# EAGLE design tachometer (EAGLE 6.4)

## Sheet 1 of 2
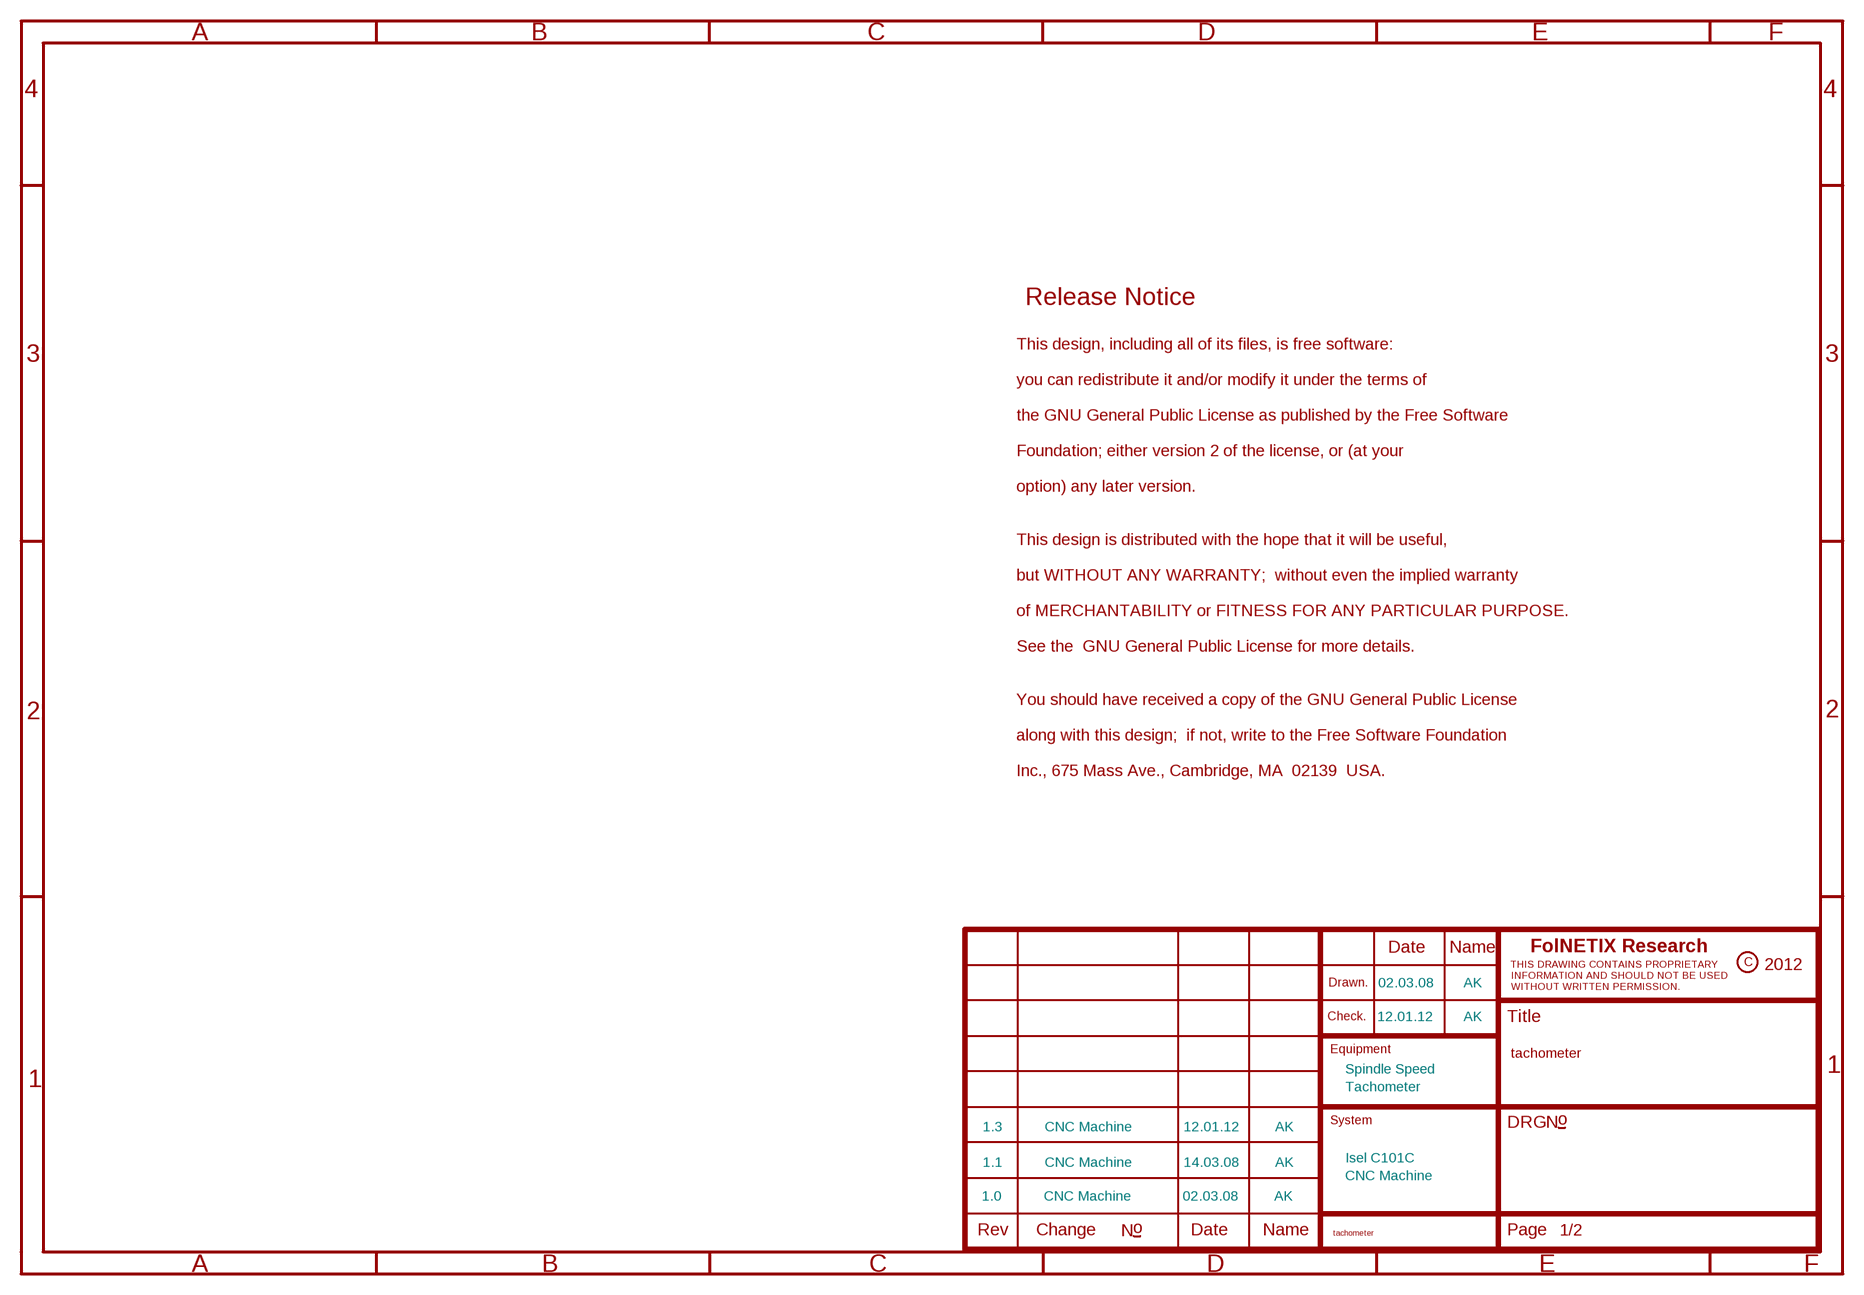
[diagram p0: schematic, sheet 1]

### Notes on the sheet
- 02.03.08 | AK
- 12.01.12 | AK
- Spindle Speed
- Tachometer
- 1.3 | CNC Machine | 12.01.12 | AK
- Isel C101C
- 1.1 | CNC Machine | 14.03.08 | AK
- CNC Machine
- 1.0 | CNC Machine | 02.03.08 | AK

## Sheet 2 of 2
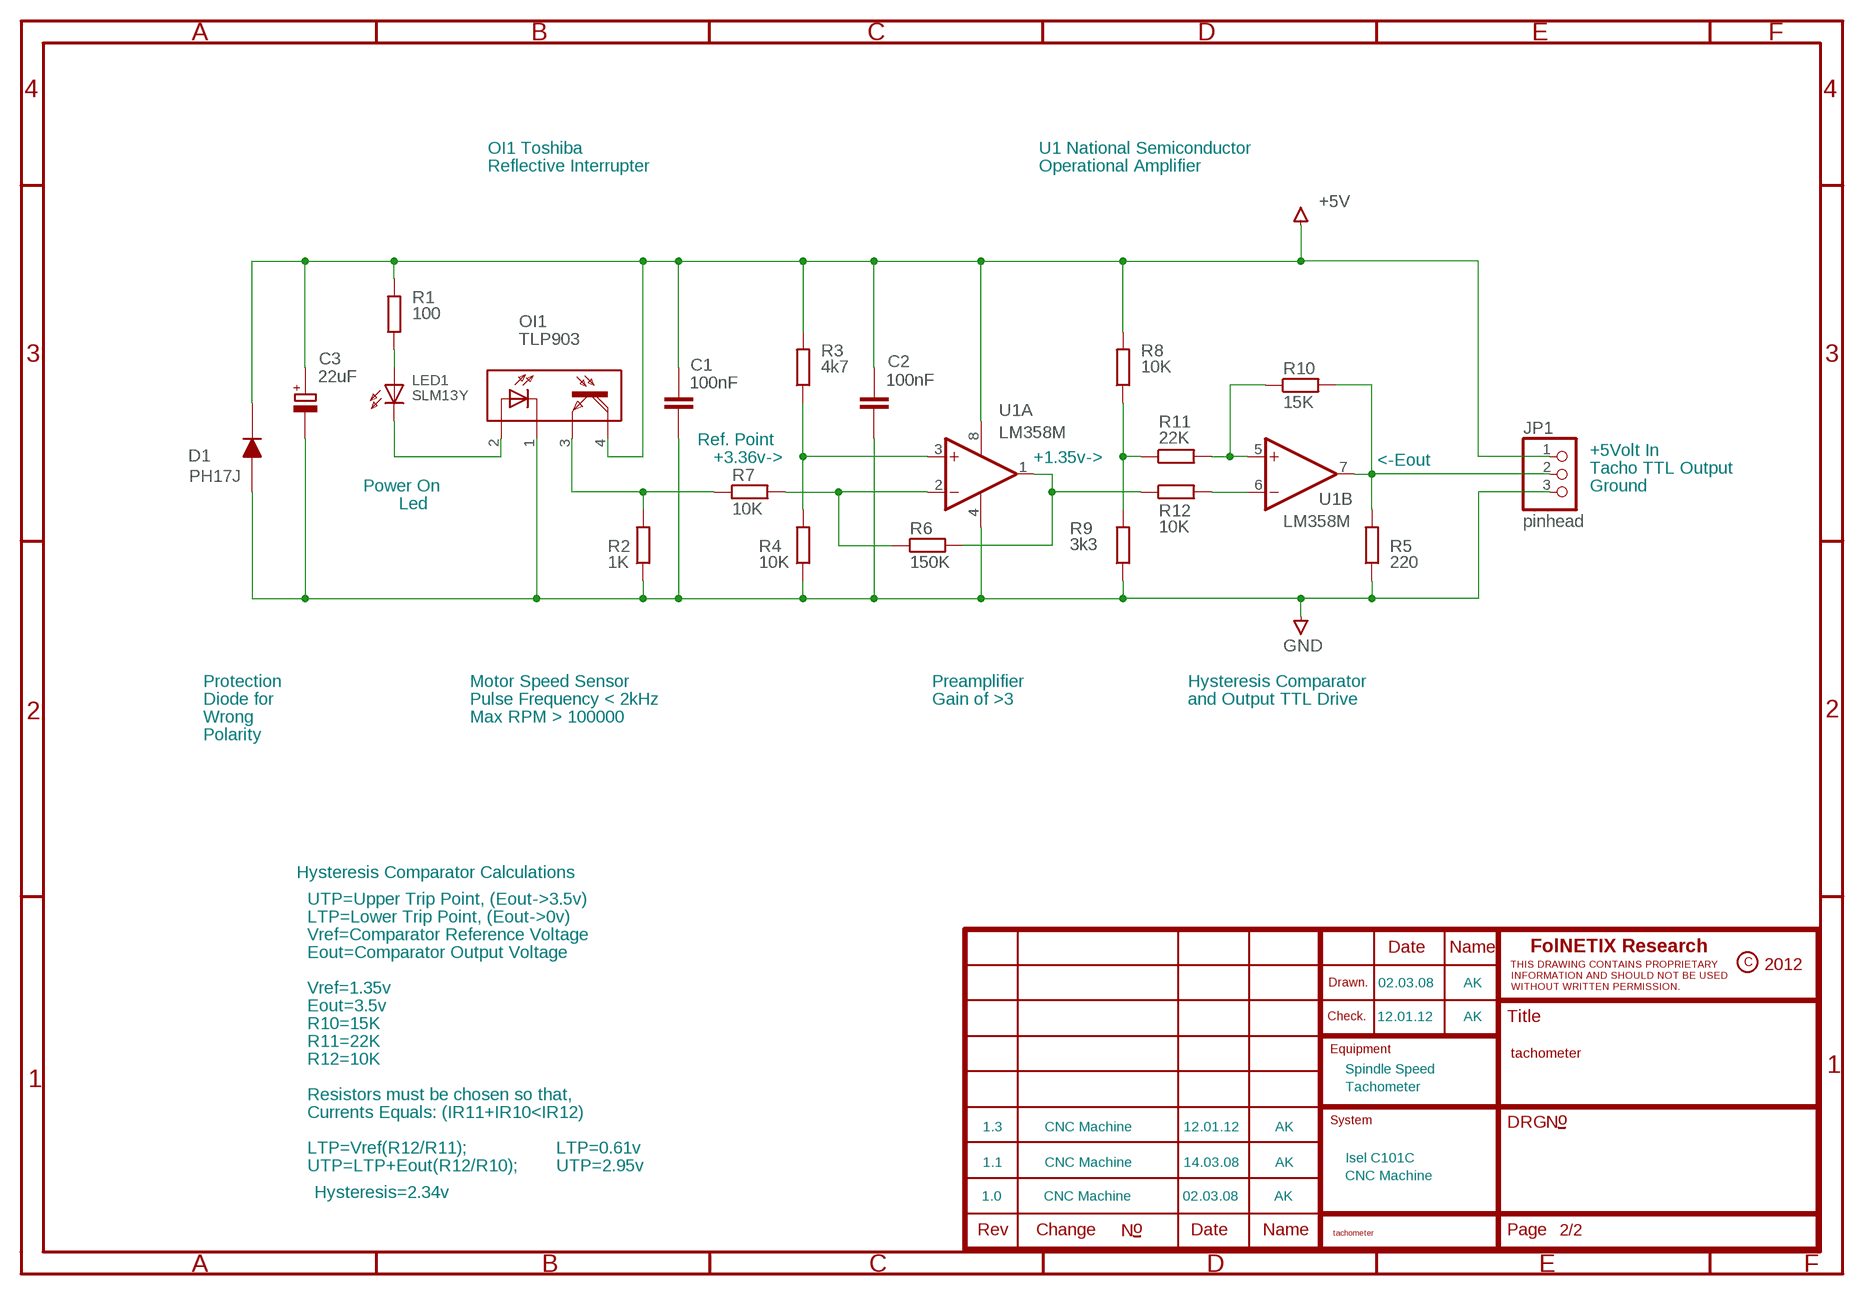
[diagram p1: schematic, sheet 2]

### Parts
C1  100nF  CAPACITOR_0603  [CAPC1608X92N]
C2  100nF  CAPACITOR_0603  [CAPC1608X92N]
C3  22uF  POLARISED_B_CASE  [CAPMP3528X210N]
D1  PH17J  [MELF]
JP1  pinhead  PINHD-1X3M  [1X03M]
LED1  SLM13Y  [SOT23_LED]
OI1  TLP903  [GAP-1E]
R1  100  RESISTOR_0603  [RESC1608X55N]
R2  1K  RESISTOR_0603  [RESC1608X55N]
R3  4k7  RESISTOR_0603  [RESC1608X55N]
R4  10K  RESISTOR_0603  [RESC1608X55N]
R5  220  RESISTOR_0603  [RESC1608X55N]
R6  150K  RESISTOR_0603  [RESC1608X55N]
R7  10K  RESISTOR_0603  [RESC1608X55N]
R8  10K  RESISTOR_0603  [RESC1608X55N]
R9  3k3  RESISTOR_0603  [RESC1608X55N]
R10  15K  RESISTOR_0603  [RESC1608X55N]
R11  22K  RESISTOR_0603  [RESC1608X55N]
R12  10K  RESISTOR_0603  [RESC1608X55N]
U1  LM358M  [SO8]

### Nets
+5V: C1.2 C2.2 C3.+ D1.2(C) JP1.1 OI1.4(TC) R1.2 R3.2 R8.2 U1.8(A:V+)
GND: C1.1 C2.1 C3.- D1.1(A1) JP1.3 OI1.1(LC) R2.1 R4.1 R5.1 R9.1 U1.4(A:V-)
N$1: LED1.3(K) OI1.2(LA)
N$2: OI1.3(TE) R2.2 R7.1
N$3: R3.1 R4.2 U1.3(A:+IN)
N$4: LED1.1(A) R1.1
N$6: JP1.2 R5.2 R10.2 U1.7(B:OUT)
N$7: R6.2 R12.1 U1.1(A:OUT)
N$8: R6.1 R7.2 U1.2(A:-IN)
N$9: R8.1 R9.2 R11.1
N$10: R10.1 R11.2 U1.5(B:+IN)
N$11: R12.2 U1.6(B:-IN)

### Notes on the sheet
- OI1 Toshiba | U1 National Semiconductor
- Reflective Interrupter | Operational Amplifier
- Ref. Point
- +5Volt In
- +3.36v-> | +1.35v-> | <-Eout
- Tacho TTL Output
- Power On | Ground
- Led
- Protection | Motor Speed Sensor | Preamplifier | Hysteresis Comparator
- Diode for | Pulse Frequency < 2kHz | Gain of >3 | and Output TTL Drive
- Wrong | Max RPM > 100000
- Polarity
- Hysteresis Comparator Calculations
- UTP=Upper Trip Point, (Eout->3.5v)
- LTP=Lower Trip Point, (Eout->0v)
- Vref=Comparator Reference Voltage
- Eout=Comparator Output Voltage
- 02.03.08 | AK
- Vref=1.35v
- Eout=3.5v
- 12.01.12 | AK
- R10=15K
- R11=22K
- R12=10K
- Spindle Speed
- Tachometer
- Resistors must be chosen so that,
- Currents Equals: (IR11+IR10<IR12)
- 1.3 | CNC Machine | 12.01.12 | AK
- LTP=Vref(R12/R11); | LTP=0.61v
- Isel C101C
- 1.1 | CNC Machine | 14.03.08 | AK
- UTP=LTP+Eout(R12/R10); | UTP=2.95v
- CNC Machine
- Hysteresis=2.34v | 1.0 | CNC Machine | 02.03.08 | AK

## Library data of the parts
C1 C2 = ipc-7351-capacitor:CAPACITOR_
C3 = ipc-7351-capacitor:POLARISED_
D1 = diode_mpad:PH17J
JP1 = pinhead_extra:PINHD-1X3: PIN HEADER
LED1 = user1:SLM13Y
OI1 = misc_opto:TLP903
R1-R12 = ipc-7351-resistor:RESISTOR_
U1 = user1:LM358M

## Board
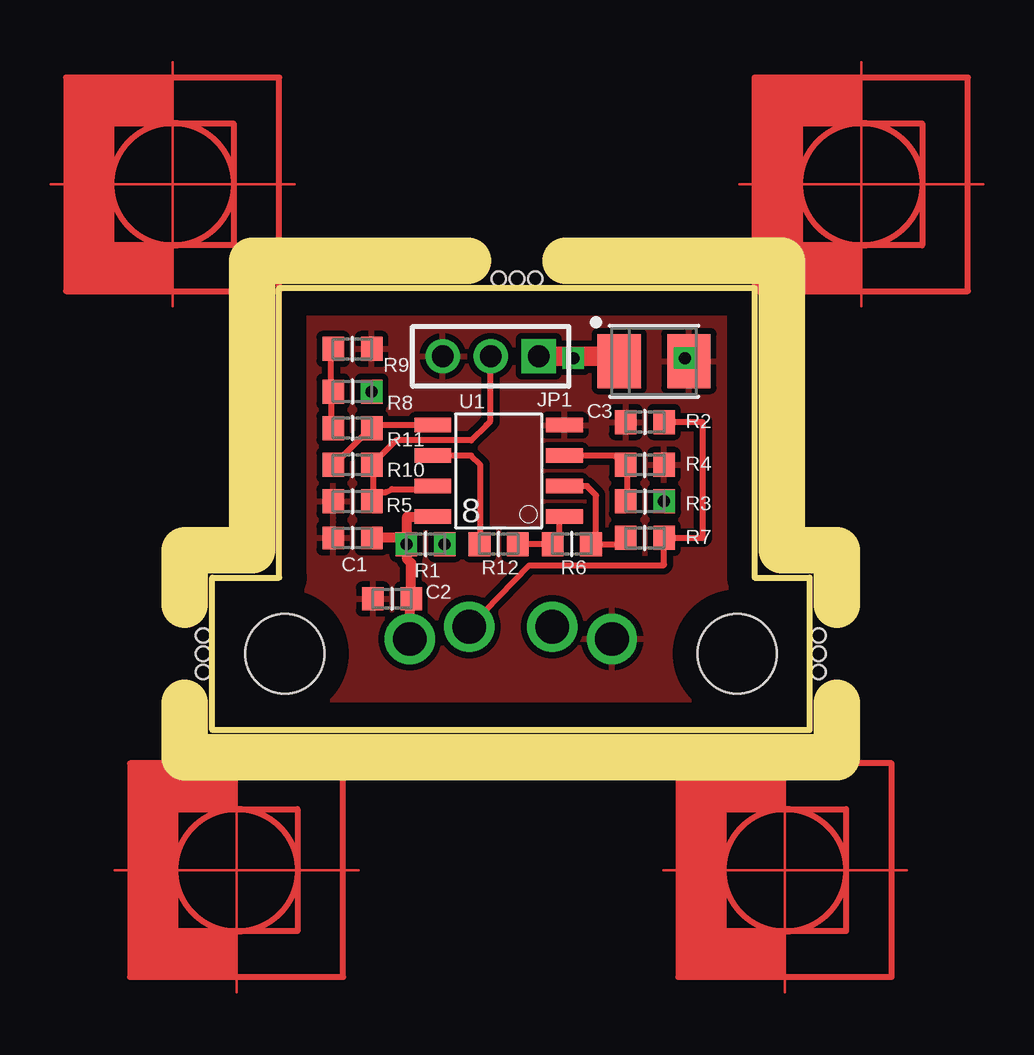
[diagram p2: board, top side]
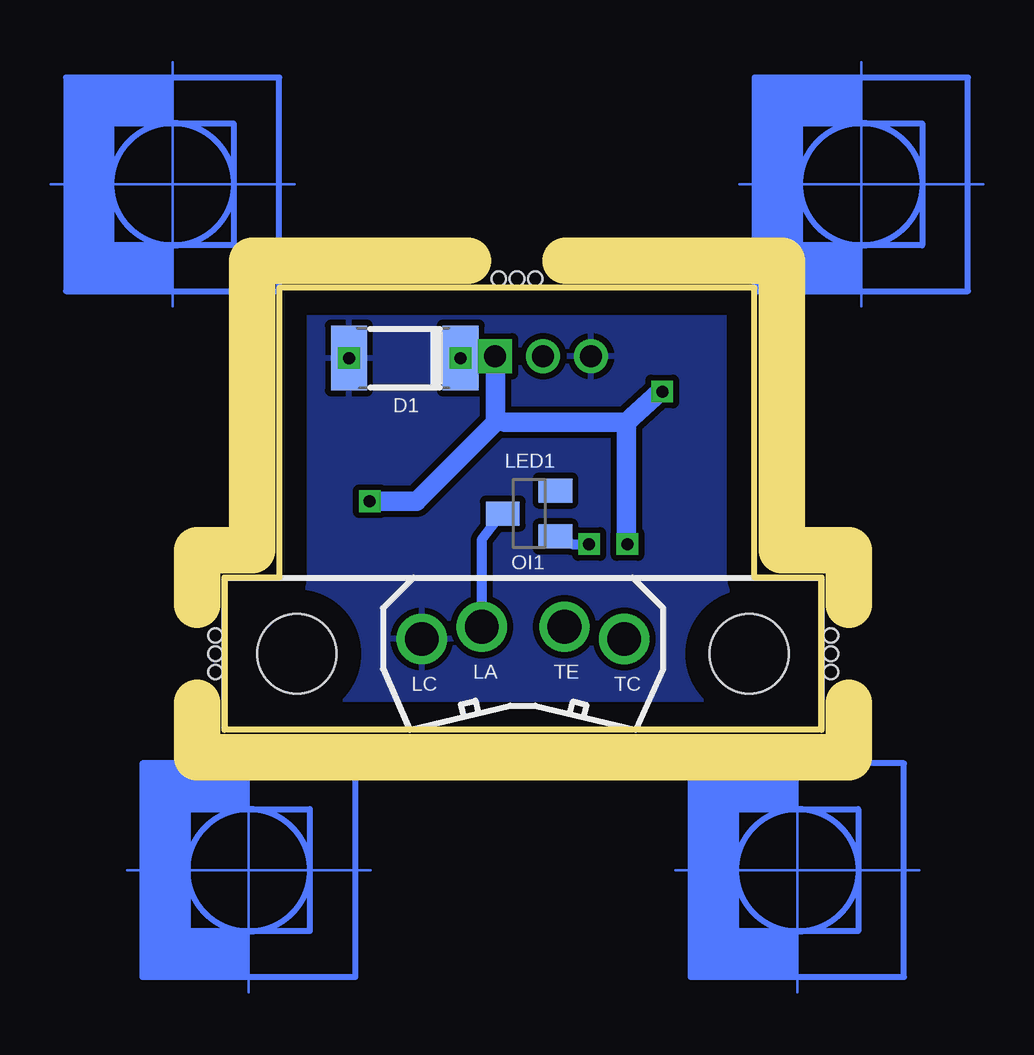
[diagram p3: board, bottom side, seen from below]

Size 24.89 x 18.42 mm. Coordinates in mm from the lower left corner, seen from the top.
Outline: 0,0 0,6.35 2.79,6.35 2.79,18.42 22.61,18.42 22.61,6.35 24.89,6.35 24.89,0 0,0
Copper layers (1*16): Top 0.035mm / dielectric 1.5mm / Bottom 0.035mm
Design rules "default": minimum track width 10mil, minimum drill 24mil, track to track 10mil, track to pad 10mil, pad to pad 10mil, via to via 10mil, smd to smd 10mil, copper to edge 40mil, drill to drill 8mil, minimum pad ring 10mil, minimum via ring 8mil, stop-mask expansion 4mil, vias tented up to drill 0mil, thermal gap 10mil
Holes 0.5 mm at 67.61,6.1
Holes 0.91 mm at 67.61,1.02
Holes 1.4 mm at 67.61,-4.06
Holes 3.3 mm at 67.61,-9.14
Holes 0.6 mm at 11.94,18.8 12.7,18.8 13.46,18.8 25.27,2.41 25.27,3.17 25.27,3.94 -0.38,2.41 -0.38,3.17 -0.38,3.94
tRestrict: area -71.8,-9 to -71,-8.5; area -74,-24 to -71.5,-21.1; area -57.8,-24.1 to -55.2,-21.2
bRestrict: area -74,-24 to -71.5,-21.1; area -57.8,-24.1 to -55.2,-21.2
Milling: 11 lines

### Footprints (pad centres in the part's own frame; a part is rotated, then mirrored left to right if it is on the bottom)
CAPC1608X92N = smd 0.9 x 0.95: 1 -0.8,0; 2 0.8,0
CAPMP3528X210N = smd 1.8 x 2.25: + -1.45,0; - 1.45,0
MELF = smd 1.5 x 2.7: 1 -2.3,0; 2 2.35,0
1X03M = drill 0.914 square: 1 -2,0 | drill 0.914: 2 0,0; 3 2,0
SOT23_LED = smd 1 x 1.4: 1 -0.95,-1.1; 2 0.95,-1.1; 3 0,1.1
GAP-1E = drill 1.4: 1 -4.216,0.744; 2 -1.727,1.252; 3 1.727,1.252; 4 4.216,0.744 | hole 3.3: 9.427,0.127; -9.427,0.127
RESC1608X55N = smd 0.9 x 1: 1 -0.8,0; 2 0.8,0
SO8 = smd 0.61 x 1.524: 1 -1.905,-2.743; 2 -0.635,-2.743; 3 0.635,-2.743; 4 1.905,-2.743; 5 1.905,2.743; 6 0.635,2.743; 7 -0.635,2.743; 8 -1.905,2.743

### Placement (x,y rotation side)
C1  5.84,8 0 top
C2  7.49,5.46 0 top
C3  18.41,15.37 0 top
D1  17.4,15.49 0 bottom
JP1  11.61,15.57 180 top
LED1  12.19,9.02 90 bottom
OI1  12.45,3.05 0 bottom
R1  8.89,7.75 180 top
R2  18.03,12.83 0 top
R3  18.03,9.53 0 top
R4  18.03,11.05 180 top
R5  5.84,9.53 0 top
R6  14.99,7.75 180 top
R7  18.03,8 180 top
R8  5.84,14.1 0 top
R9  5.84,15.88 180 top
R10  5.84,11.05 0 top
R11  5.84,12.57 0 top
R12  11.94,7.75 180 top
U1  11.94,10.8 90 top
U$1  [FAB_DOCFIELD]  not placed on the board
U$2  [PASSMARK]  not placed on the board
U$3  [PASSMARK]  not placed on the board
U$4  [PASSMARK]  not placed on the board
U$5  [PASSMARK]  not placed on the board
U$6  [FAB_TABL_L]  not placed on the board

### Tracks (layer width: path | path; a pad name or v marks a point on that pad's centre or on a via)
+5V  (via drill 0.5)
  Top 0.254: R8.2 | 6.73,8 C1.2 6.57,8 | 7.87,8 R1.2 8.13,7.75 | 8.76,8.89 U1.8 | 16.51,15.57 16.51,15.62 16.26,15.37 D1.2
  Top 0.406: 16.51,15.57 C3.+ | 7.87,8 C1.2 | 8.76,8.89 8.13,8.89 8.13,7.75 8.13,7.11 8.29,6.95 C2.2 | C2.2 8.23,5.46 | C2.2 8.23,5.46 | 8.23,5.46 OI1.4 | OI1.4 | OI1.4
  Top 0.813: JP1.1 16.51,15.57
  Bottom 0.406: 13.59,15.49 13.61,15.51 | 6.73,14.1 R8.2 | 13.21,12.83 13.59,12.83 | R1.2 8.13,7.75 8.13,7.87
  Bottom 0.813: R3.2 16.89,9.53 13.59,12.83 13.59,15.49 | 13.61,15.51 JP1.1 | 8.13,12.83 6.73,14.1 | 8.13,12.83 13.21,12.83 | 8.13,7.87 8.13,12.83
  other vias: 18.83,9.53 6.64,14.1 8.09,7.75 15.05,15.49
GND  (via drill 0.5)
  other vias: 19.7,15.49
  pour Top: 3.05,18.03 22.48,18.03 22.48,0 3.05,0
  pour Bottom: 3.05,18.03 22.48,18.03 22.48,0 3.05,0
N$1
  Bottom 0.406: LED1.3 13.33,9.02 14.17,7.92 OI1.2
N$2
  Top 0.254: R2.2 20.45,12.83 20.45,8 R7.1 | R7.1 18.8,8 | R7.1 18.83,6.9 18.8,6.86 13.21,6.86 OI1.3
  Top 0.406: OI1.3
N$3
  Top 0.254: R3.1 17.27,9.54 17.3,11.05 R4.2 16.76,11.43 U1.3
  Top 0.406: R4.2
N$4  (via drill 0.5)
  Bottom 0.406: LED1.1 11.18,8.07 11.18,8 10.41,7.75 R1.1
  other vias: 9.69,7.75
N$6
  Top 0.25: 11.43,12.7 10.79,12.06 7.66,12.06 R10.2
  Top 0.254: 6.62,9.54 6.71,9.53 6.73,9.53 | U1.7 8.64,10.03 7.49,10.03 7.24,9.91 6.98,9.91 6.73,9.53 | JP1.2 11.6,12.87 11.43,12.7 | R10.2 6.58,11.05 | 6.73,9.53 6.73,11.05
  Top 0.406: R5.2 6.73,9.53 | 6.73,11.05 R10.2
N$7
  Top 0.25: R6.2 R12.1
  Top 0.254: R12.1 12.7,7.75 | 14.22,7.75 R6.2 14.48,8.01 14.48,8.89 U1.1
N$8
  Top 0.254: 17.3,8 R7.2 17.02,7.87 17.02,7.75 R6.1 15.75,7.75 16,8 16,9.78 15.62,10.16 U1.2
N$9
  Top 0.254: R9.2 4.95,15.88 4.95,14.1 | R11.1 4.95,12.57 4.95,14.1 | R8.1 4.95,14.1
N$10
  Top 0.25: U1.5 6.73,12.7 5.08,11.05
  Top 0.406: 6.73,12.7 6.64,12.7 R11.2 | R11.2 | R11.2 | R11.2 | R11.2 | 5.08,11.05 R10.1
N$11
  Top 0.254: U1.6 10.79,11.43 11.18,11.05 11.18,8 R12.2

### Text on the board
Holes: (Set the drill symbols with | Options - Set - Drill - Set) | Drill file will contain one extra of | each drill, placed in above diagram. | DRILL PLAN | SYM | SIZE | TOL. | CNT | PLATE | 0.50 mm | +/-0.08 mm | 6 | Yes | 0.91 mm | +/-0.08 mm | 3 | Yes | 1.40 mm | +/-0.08 mm | 4 | Yes | 3.30 mm | +/-0.08 mm | 2 | 0 | TOTAL | 15 | 13
Document: FABRICATION DRAWING | NOTES: | 1. PRINTED CIRCUIT BOARD MADE FROM NEMA GRADE FR-4 EPOXY LAMINATE | WITH 1 OUNCE COPPER PLATING AND 1.6mm THICKNESS. | 2. ALL DIMENSIONS ARE GIVEN IN MILLIMETERS. | 3. CIRCUIT PATHS ARE FOR REFERENCE ONLY. | 4. HOLE SIZES SHOWN ARE FINISHED DIAMETERS BEFORE PLATING. | 5. BOARD PLATED USING REFLOW OR SIMILAR METHOD. | 6. BOARD TO HAVE GREEN SOLDER MASK ON PLATED SURFACES USING WET FILM | SR100 OR SR1010 EPOXY. EQUIVALENT WET OR DRY FILM MAY BE USED. | 7. SILKSCREEN BOARD USING YELLOW INK. | 8. THE FOLLOWING INFORMATION APPLIES TO THIS BOARD: | * 2 COPPER LAYERS | * 1.6mm BOARD THICKNESS | * REQUIRES TOP AND BOTTOM SIDE SILKSCREEN | (Set the drill symbols with | Options - Set - Drill - Set) | Drill file will contain one extra of | each drill, placed in above diagram. | DRILL PLAN | SYM | SIZE | TOL. | CNT | PLATE | 0.50 mm | +/-0.08 mm | 6 | Yes | 0.91 mm | +/-0.08 mm | 3 | Yes | 1.40 mm | +/-0.08 mm | 4 | Yes | 3.30 mm | +/-0.08 mm | 2 | 0 | TOTAL | 15 | 13
Infotext: Transistor / Collector | Transistor / Emitter | Diode / Anode | Diode / Cathode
